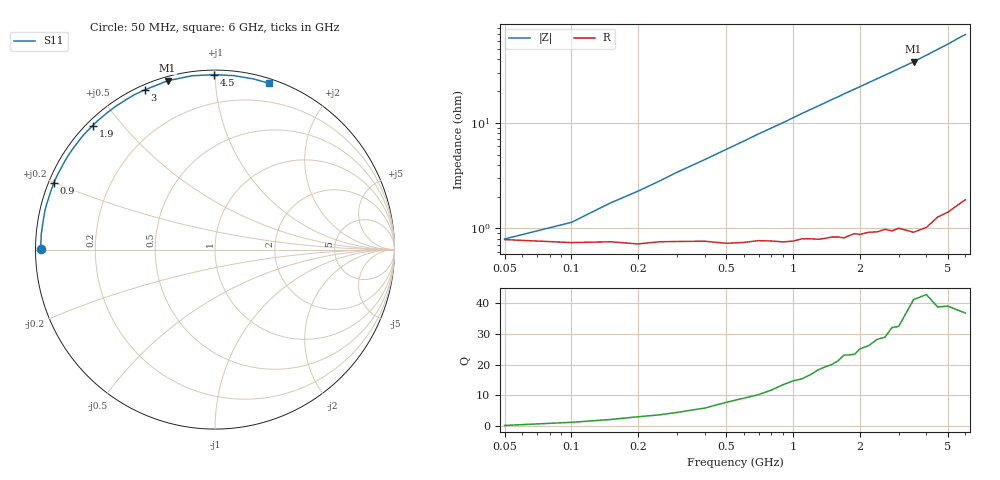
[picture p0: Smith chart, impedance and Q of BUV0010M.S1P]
! Infineon Technologies  Discrete & RF Semiconductors
! BB 833
! Si Tuning Diode in SOD323
! VR =
! S-Parameters:  June  1999
# GHz  S  MA  R  50
!  f  S11
! GHz  MAG  ANG
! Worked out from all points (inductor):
!   34 points, 50 MHz to 6 GHz, reference 50 ohm
!   read as one part to ground: L = 1.72 nH near 200 MHz
!   highest Q = 41.2 at 3.5 GHz (marker M1), where L = 1.72 nH
!   S11 on the Smith chart (normalised r, x): 50 MHz: 0.02, +0.00; 900 MHz: 0.01, +0.20; 1.9 GHz: 0.02, +0.42; 3 GHz: 0.02, +0.65; 4.5 GHz: 0.03, +0.99; 6 GHz: 0.04, +1.38
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0.05  0.9692 179.7
0.1  0.9711 178.0
0.15  0.9706 176.4
0.2  0.972 175.1
0.3  0.9706 172.4
0.5  0.9719 167.3
0.7  0.9706 162.2
0.8  0.971 159.8
0.9  0.9718 157.4
1.1  0.9704 152.4
1.2  0.9707 150.1
1.4  0.9711 145.5
1.5  0.9706 143.2
1.6  0.971 141.1
1.7  0.9719 138.8
1.9  0.9701 134.6
2  0.9711 132.6
2.2  0.9706 128.5
2.4  0.9713 124.7
2.6  0.9708 120.9
2.8  0.9728 117.4
3  0.9722 113.8
3.5  0.9769 105.7
4  0.9772 97.6
4.5  0.9746 90.3
5  0.9749 83.8
5.5  0.9746 77.4
6  0.9745 72.0
